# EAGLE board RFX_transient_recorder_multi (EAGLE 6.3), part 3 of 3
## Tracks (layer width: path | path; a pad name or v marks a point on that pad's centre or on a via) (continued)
N$84 (continued)
  Top 0.254: C72.2 52.8,19.14 55.9,19.14 55.9,20.14 56.1,20.34 57.7,20.34 57.7,19.04 IC4.2 57.8,18.94 R44.1 57.8,6.34 60.3,3.84 R43.2
N$85
  Top 0.254: R45.2 24.8,3.74 25.5,3.04 29.8,3.04 29.8,3.74 U2.1
N$86  (via drill 0.61 layers 1-2)
  Top 0.254: v33,6.84 29.1,6.84 26.1,3.84 R45.1 | v34.6,8.44 37,10.84 42,10.84 42,9.94 42.2,9.74 42.8,9.74 U1.22
  top_internal 0.254: v34.6,8.44 v33,6.84
N$87
  Top 0.254: R46.1 38.8,10.14 39.7,9.24 42.8,9.24 U1.23
N$88
  Top 0.254: 36.8,7.54 36.8,9.54 37.4,10.14 R46.2 | 36.8,7.54 36.8,4.44 37.4,3.84 R47.2 | 36.8,7.54 33.3,7.54 33.1,7.74 33.1,8.24 32.4,8.94 U2.6
N$89
  Top 0.254: R47.1 38.8,3.84 39,4.04 39,4.94 40.5,6.44 46.2,6.44 46.2,7.24 U1.29
N$90
  Top 0.254: U2.2 31.2,3.84 32.3,3.84 U2.3
N$91  (via drill 0.61 layers 1-2)
  Top 0.254: v40.6,11.84 36.5,11.84 33.7,9.04 U2.5 | v75.3,9.14 78.8,9.14 78.8,13.24 79,13.44 90.1,13.44 U3.2
  top_internal 0.254: v40.6,11.84 40.8,11.64 61.9,11.64 63.8,9.74 74.7,9.74 v75.3,9.14
N$92
  Top 0.254: R48.1 38.8,6.44 39.9,6.44 41.7,8.24 43.8,8.24 43.8,9.94 43.6,10.14 42.9,10.14 U1.21
N$93  (via drill 0.61 layers 1-2)
  Top 0.254: v38,7.44 38,6.94 37.5,6.44 R48.2 | v74.5,7.44 78.5,7.44 80.6,9.54 88.7,9.54 88.7,11.14 89.6,12.04 90.1,12.04 U3.3
  top_internal 0.254: v74.5,7.44 v38,7.44
N$94  (via drill 0.61 layers 1-2)
  Top 0.254: 55.9,4.94 55.9,3.34 55.4,2.84 50.7,2.84 50.7,5.74 50,6.44 49.3,6.44 49.3,7.24 U1.35 | 55.9,4.94 55.9,5.74 56.5,6.34 C74.2 | v75.3,5.64 78.6,5.64 79.3,6.34 R49.2 | 55.9,4.94 v56.6,4.94
  top_internal 0.254: v75.3,5.64 74.6,4.94 v56.6,4.94
N$95
  Top 0.254: R49.1 78.1,6.44 78.8,7.14 88.7,7.14 88.7,6.64 89.6,5.74 90.1,5.74 U16.6
N$96  (via drill 0.61 layers 1-2)
  Top 0.254: v48.3,5.84 48.7,6.24 48.7,7.24 U1.34 | v63,3.84 65,1.84 88.7,1.84 88.7,3.54 89.6,4.44 U16.7
  top_internal 0.254: v48.3,5.84 50.3,3.84 v63,3.84
N$97  (via drill 0.61 layers 1-2)
  Top 0.254: v103.8,8.54 103.8,9.94 99.8,13.94 R50.2 | v106.3,6.04 105.1,6.04 U17.5
  top_internal 0.254: v106.3,6.04 v103.8,8.54
N$98
  Top 0.254: R51.2 103.7,7.44 103.7,5.24 104.2,4.74 105,4.74 U17.7
N$99  (via drill 0.61 layers 1-2)
  Top 0.254: v98.4,12.84 98.4,13.94 R50.1 | v93.6,12.84 95.3,12.84 95.3,13.24 U3.7
  top_internal 0.254: v93.6,12.84 v98.4,12.84
N$100  (via drill 0.61 layers 1-2)
  Top 0.254: v98.4,10.34 98.4,11.34 R51.1 | v96.8,9.94 96.7,10.04 96.7,11.14 95.8,12.04 95.4,12.04 U3.6
  top_internal 0.254: v98.4,10.34 98,9.94 v96.8,9.94
N$101  (via drill 0.61 layers 1-2)
  Top 0.254: v113.8,2.54 R52.2 | v112.1,3.34 111.4,4.04 110.9,4.04 U17.9
  top_internal 0.254: v113.8,2.54 113,3.34 v112.1,3.34
N$102
  Top 0.254: 113.1,5.64 116.2,2.54 R52.1 | 113.1,5.64 113.1,10.84 111.9,12.04 U18.1 | U16.3 95.3,5.64 93.9,5.64 93.9,2.84 94.4,2.34 113,2.34 113,5.64 113.1,5.64
N$103  (via drill 0.61 layers 1-2)
  Top 0.254: v107.1,19.04 103.6,19.04 R53.1 | v96.8,7.84 96.8,4.54 95.4,4.54 U16.2
  top_internal 0.254: 107.65,18.49 110.9,15.24 X7.8 | 107.65,18.49 v107.1,19.04 | v96.8,7.84 98.5,9.54 98.7,9.54 107.65,18.49
N$104
  Top 0.254: U18.2 111.9,13.34 111.9,14.54 U18.3
N$105  (via drill 0.61)
  Top 0.254: 104.9,14.04 106.6,14.04 106.6,14.54 U18.6 | 104.9,14.04 103.6,14.04 R54.1 | v104.9,14.14 104.9,14.04
  bottom_internal 0.254: v104.9,14.14 124.4,14.14 124.4,15.24 X7.7
N$106  (via drill 0.61 layers 1-2)
  Top 0.254: 107.9,24.34 107.9,16.34 108,16.24 108,13.44 107.25,12.69 | 107.9,24.34 107.9,24.74 108.5,25.34 C81.2 | 107.25,12.69 106.7,12.14 U18.8 | v110.9,25.34 112,25.34 U19.5 | v108,24.34 107.9,24.34 | 107.25,12.69 106.7,13.24 U18.7
  top_internal 0.254: v110.9,25.34 109.9,24.34 v108,24.34
N$107  (via drill 0.61 layers 1-2)
  Top 0.254: v117.5,24.34 117.5,25.34 C82.2 | v114.8,24.54 114,25.34 U19.4
  top_internal 0.254: v117.5,24.34 117.3,24.54 v114.8,24.54
N$108  (via drill 0.61 layers 1-2)
  Top 0.254: v74.9,12.84 74.9,9.94 77.4,9.94 77.6,10.14 78,10.14 C54.1 | v66.8,20.94 64.8,20.94 64.8,20.04 U20.4
  top_internal 0.254: v66.8,20.94 v74.9,12.84
N$109  (via drill 0.61 layers 1-2)
  Top 0.254: v77.1,10.74 77.1,11.74 78,12.64 C55.1 | v67.6,10.64 66.1,10.64 66.1,9.84 U21.4
  top_internal 0.254: v77.1,10.74 77,10.64 v67.6,10.64
N$110
  Top 0.254: C56.1 49,24.14 49.3,24.44 49.3,25.74 49.5,25.94 64.7,25.94 64.7,25.14 U22.4
N$111
  Top 0.254: C57.1 73,8.84 69.9,5.74 69.9,2.74 69.5,2.34 65.1,2.34 65.1,3.84 66,4.74 U23.4
N$112  (via drill 0.61 layers 1-2)
  Top 0.254: v100.3,15.94 106.6,15.94 U18.5
  top_internal 0.254: v100.3,15.94 99.8,16.44 97.8,16.44 U24.P$14
N$115  (via drill 0.61 layers 1-2)
  Top 0.254: X6.9 24.1,17.84 24.1,20.24 X6.10 | U24.P$7 82.5,24.04 79.8,21.34 73.4,21.34 73.4,20.44 C2.1.- 73.4,20.24 72.2,19.04 72.2,14.94 69.6,14.94 69.5,14.84 68.8,14.84 IC3.3 68.7,14.84 68.7,14.04 IC3.2 68.8,14.04 69.5,13.34 69.5,12.04 v62.6,12.04
  top_internal 0.254: v62.6,12.04 58.4,12.04 53.9,16.54 25.4,16.54 24.2,17.74 X6.9
N$116  (via drill 0.61 layers 1-2)
  Top 0.254: X6.7 21.6,17.84 21.6,20.24 X6.8 21.7,20.34 26.6,25.24 v48.5,25.24 | U23.1 68.7,2.94 69.5,2.94 69.5,4.14 68.9,4.74 68.7,4.74 U23.3 68.7,4.84 68.7,7.94 U21.1 68.8,7.84 69.5,8.54 69.5,9.84 | 69.5,9.84 U21.3 | 68.2,18.14 67.4,18.14 U20.1 | 68.2,18.14 68.2,19.44 67.7,19.94 67.4,19.94 U20.3 67.7,20.04 67.7,22.44 | 67.7,22.44 67.7,22.84 67.4,23.14 U22.1 67.6,23.04 68.2,23.64 68.2,24.14 | 68.2,24.14 68.2,25.04 67.4,25.04 U22.3 | 68.2,24.14 73.4,24.14 C59.+ 73.5,24.24 73.5,25.74 83.4,25.74 85,24.14 U24.P$6 | v69.9,14.14 69.9,10.34 69.5,9.94 69.5,9.84 | v69.9,15.74 68.2,17.44 68.2,18.14 | 67.7,22.44 v60.4,22.44
  top_internal 0.254: v69.9,15.74 v69.9,14.14 | v48.5,25.24 51,22.74 60.1,22.74 v60.4,22.44
N$117  (via drill 0.61 layers 1-2)
  Top 0.254: v109.6,5.34 110.8,5.34 U17.11
  top_internal 0.254: v109.6,5.34 110.3,6.04 122.9,6.04 124.4,7.54 X7.1
N$118  (via drill 0.61 layers 1-2)
  Top 0.254: v112.3,6.84 112.3,6.04 110.9,6.04 U17.12
  top_internal 0.254: v112.3,6.84 113,7.54 121.9,7.54 X7.2
N$119  (via drill 0.61 layers 1-2)
  Top 0.254: v109.6,6.54 109.6,6.64 110.8,6.64 U17.13
  top_internal 0.254: v109.6,6.54 112.2,9.14 123.4,9.14 124.4,10.14 X7.3
N$120  (via drill 0.61 layers 1-2)
  Top 0.254: v109.3,7.74 109.3,7.34 110.8,7.34 U17.14
  top_internal 0.254: v109.3,7.74 111.7,10.14 121.9,10.14 X7.4
N$121  (via drill 0.61 layers 1-2)
  Top 0.254: v110,10.94 110,8.04 110.8,8.04 U17.15
  top_internal 0.254: v110,10.94 112.8,13.74 123.4,13.74 124.4,12.74 X7.5
N$122  (via drill 0.61)
  Top 0.254: v112.3,8.14 112.3,8.54 110.9,8.54 U17.16
  bottom_internal 0.254: v112.3,8.14 116.8,12.64 121.9,12.64 X7.6
N$123
  Top 0.254: R62.2 4.4,50.8 3.2,52 3.2,53.3 C86.1 3.2,53.4 3.2,55 5.3,57.1 L5.2
N$124
  Top 0.254: R58.1 3.2,64.7 3.2,61 C85.1 3.1,60.9 3.1,57.9 2.4,57.2 L5.1
N$125
  Top 0.254: C86.2 4.5,53.3 9.5,53.3 R63.2 9.6,53.4 9.6,55.1 11.6,57.1 L6.2
N$126
  Top 0.254: C85.2 4.5,61 8.2,61 R59.1 8.3,60.9 8.3,57.5 8.6,57.2 L6.1
N$127
  Top 0.254: 14.6,50.1 16.4,50.1 16.5,50.2 16.5,59.4 18.8,59.4 U$3.11 | 14.6,50.1 R65.1 14.6,50.9 14.6,53.3 R66.2 14.6,53.4 14.6,57.1 C87.1 | 14.6,50.1 3.9,50.1 3.2,50.8 R62.1
N$128  (via drill 0.61, 0.61 layers 1-2)
  Top 0.254: R64.1 10.8,53.3 R63.1 10.9,53.4 v13.7,56.2 | 23.8,59.4 24.2,59.4 24.2,59 24.7,58.5 R67.2 | 23.8,59.4 21.8,59.4 U$3.2 | v31.9,64 31.9,65.5 32.4,66 C88.1 | 23.8,59.4 v23.8,59.1
  top_internal 0.254: v13.7,56.2 16.6,59.1 v23.8,59.1
  bottom_internal 0.254: v31.9,64 27,59.1 v23.8,59.1
N$129
  Top 0.254: X8.3 16.5,66 14.8,64.3 14.8,62.4 13.4,61 R57.2 13.3,60.9 13.3,60.2 9.1,60.2 8.9,60.4 8.9,61.7 7.5,61.7 4.5,64.7 R58.2
N$130
  Top 0.254: R59.2 9.6,61 12,61 R57.1 12,61.1 14.4,63.5 14.4,65 15.5,66.1 15.5,67.5 16.5,68.5 X8.4
N$131
  Top 0.254: R66.1 15.9,53.4 15.9,57.1 C87.2 15.9,57.2 15.9,60 | 15.9,60 18.8,60 U$3.10 | 15.9,60 15.9,60.9 R68.2
N$132  (via drill 0.61 layers 1-2)
  Top 0.254: C88.2 31.1,63.1 | 31.1,63.1 R69.2 | 26.7,62.8 25,62.8 24,61.8 24,59.9 21.8,59.9 U$3.3 | 26.7,62.8 26.7,60.4 26.1,59.8 26.1,58.5 R67.1 | v30.3,63.1 31.1,63.1 | v28.3,63 26.7,63 26.7,62.8
  top_internal 0.254: v30.3,63.1 30.2,63 v28.3,63
N$133  (via drill 0.61 layers 1-2)
  Top 0.254: R68.1 18,61.8 v18,62 | v25.3,62 26,61.3 26,61 C89.2 | v52.3,57.9 51.1,57.9 U25.39
  top_internal 0.254: v18,62 v25.3,62 26.1,62 28.8,59.3 50.9,59.3 v52.3,57.9
N$134  (via drill 0.61)
  Top 0.254: R69.1 32.4,60.9 | 32.4,60.9 32.4,59 31.8,58.4 31.8,55.8 26.1,55.8 C90.2 | v52.3,59.1 52.3,59.9 51.1,59.9 U25.43 | 32.4,60.9 v38.6,60.9
  bottom_internal 0.254: v52.3,59.1 50.5,60.9 v38.6,60.9
N$135  (via drill 0.61 layers 1-2)
  Top 0.254: v60.7,61.1 60.7,61.9 60.4,62.2 R61.1 | v62.6,62.1 66,62.1 66,63.1 IC5.4 | v70.7,61.5 71.1,61.5 72.6,63 72.6,64.3 73,64.7 R60.1
  top_internal 0.254: v60.7,61.1 61.7,62.1 v62.6,62.1 67.4,62.1 67.9,61.6 70.6,61.6 v70.7,61.5
N$136  (via drill 0.61 layers 1-2)
  Top 0.254: IC6.6 59,72.5 57.8,72.5 IC6.7 58,72.4 58,69.9 57.1,69 50.8,69 v50.3,68.5 | v18.8,61.2 18.8,60.5 U$3.9 | v21.9,61.2 21.8,61.1 21.8,60.5 U$3.4 | 30.55,67.95 30.5,67.9 30.5,64.4 29.5,63.4 29.5,61.5 v27.5,59.5 | 30.55,67.95 31.1,68.5 C91.2 | v37.9,68.4 33,68.4 33,68 32.9,67.9 30.6,67.9 30.55,67.95
  top_internal 0.254: v18.8,61.2 v21.9,61.2 22,61.2 22.3,61.5 23.3,61.5 23.6,61.2 25.8,61.2 v27.5,59.5 | v50.3,68.5 50.2,68.4 v37.9,68.4
N$137  (via drill 0.61 layers 1-2)
  Top 0.254: v56.6,51 56.6,52 R70.2 | v58.2,51 61.6,51 61.6,52 R71.1 61.7,52.1 61.7,52.5 62.2,53 62.2,58.6 | C103.1 62.2,59.1 62.2,58.6 | v59.5,58.8 59.5,64 59.6,64.1 59.6,71.7 60.3,72.4 IC6.5 | 62.2,58.6 v61.8,58.6
  top_internal 0.254: v58.2,51 v56.6,51 | v59.5,58.8 59.7,58.6 v61.8,58.6
N$138
  Top 0.254: R70.1 55.2,52.1 52.3,52.1 C104.+ 52.3,55.7 51.1,56.9 U25.37
N$139
  Top 0.254: C105.1 55.2,62.2 52,62.2 52,61.7 51.8,61.5 51.1,61.5 U25.46
N$140  (via drill 0.61 layers 1-2)
  Top 0.254: R72.2 56.5,67.2 IC6.1 56.4,66.6 52.2,66.6 51.5,67.3 C114.1 51.3,67.3 v49.9,67.3 | 15.2,59.1 15.3,59.1 15.3,51.3 15.8,50.8 R65.2 | 15.2,59.1 14.2,59.1 13.6,58.5 13.6,57.3 10.2,53.9 10.2,51.4 9.6,50.8 R64.2 | v27.3,67.6 22.5,62.8 15.2,62.8 15.2,59.1
  top_internal 0.254: v49.9,67.3 49.6,67.6 v27.3,67.6
N$141
  Top 0.254: C114.2 52.8,67.4 55.9,67.4 55.9,68.4 56.1,68.6 57.7,68.6 57.7,67.3 IC6.2 57.8,67.2 R72.1 57.8,54.6 60.3,52.1 R71.2
N$142
  Top 0.254: R73.2 24.8,52 25.5,51.3 29.8,51.3 29.8,52 U26.1
N$143  (via drill 0.61 layers 1-2)
  Top 0.254: v33,55.1 29.1,55.1 26.1,52.1 R73.1 | v34.6,56.7 37,59.1 42,59.1 42,58.2 42.2,58 42.8,58 U25.22
  top_internal 0.254: v34.6,56.7 v33,55.1
N$144
  Top 0.254: R74.1 38.8,58.4 39.7,57.5 42.8,57.5 U25.23
N$145
  Top 0.254: 36.8,55.8 36.8,57.8 37.4,58.4 R74.2 | 36.8,55.8 36.8,52.7 37.4,52.1 R75.2 | 36.8,55.8 33.3,55.8 33.1,56 33.1,56.5 32.4,57.2 U26.6
N$146
  Top 0.254: R75.1 38.8,52.1 39,52.3 39,53.2 40.5,54.7 46.2,54.7 46.2,55.5 U25.29
N$147
  Top 0.254: U26.2 31.2,52.1 32.3,52.1 U26.3
N$148  (via drill 0.61 layers 1-2)
  Top 0.254: v40.6,60.1 36.5,60.1 33.7,57.3 U26.5 | v75.3,57.4 78.8,57.4 78.8,61.5 79,61.7 90.1,61.7 U27.2
  top_internal 0.254: v40.6,60.1 40.8,59.9 61.9,59.9 63.8,58 74.7,58 v75.3,57.4
N$149
  Top 0.254: R76.1 38.8,54.7 39.9,54.7 41.7,56.5 43.8,56.5 43.8,58.2 43.6,58.4 42.9,58.4 U25.21
N$150  (via drill 0.61 layers 1-2)
  Top 0.254: v38,55.7 38,55.2 37.5,54.7 R76.2 | v74.5,55.7 78.5,55.7 80.6,57.8 88.7,57.8 88.7,59.4 89.6,60.3 90.1,60.3 U27.3
  top_internal 0.254: v74.5,55.7 v38,55.7
N$151  (via drill 0.61 layers 1-2)
  Top 0.254: 55.9,53.2 55.9,51.6 55.4,51.1 50.7,51.1 50.7,54 50,54.7 49.3,54.7 49.3,55.5 U25.35 | 55.9,53.2 55.9,54 56.5,54.6 C116.2 | v75.3,53.9 78.6,53.9 79.3,54.6 R77.2 | 55.9,53.2 v56.6,53.2
  top_internal 0.254: v75.3,53.9 74.6,53.2 v56.6,53.2
N$152
  Top 0.254: R77.1 78.1,54.7 78.8,55.4 88.7,55.4 88.7,54.9 89.6,54 90.1,54 U28.6
N$153  (via drill 0.61 layers 1-2)
  Top 0.254: v48.3,54.1 48.7,54.5 48.7,55.5 U25.34 | v63,52.1 65,50.1 88.7,50.1 88.7,51.8 89.6,52.7 U28.7
  top_internal 0.254: v48.3,54.1 50.3,52.1 v63,52.1
N$154  (via drill 0.61 layers 1-2)
  Top 0.254: v103.8,56.8 103.8,58.2 99.8,62.2 R78.2 | v106.3,54.3 105.1,54.3 U29.5
  top_internal 0.254: v106.3,54.3 v103.8,56.8
N$155
  Top 0.254: R79.2 103.7,55.7 103.7,53.5 104.2,53 105,53 U29.7
N$156  (via drill 0.61 layers 1-2)
  Top 0.254: v98.4,61.1 98.4,62.2 R78.1 | v93.6,61.1 95.3,61.1 95.3,61.5 U27.7
  top_internal 0.254: v93.6,61.1 v98.4,61.1
N$157  (via drill 0.61 layers 1-2)
  Top 0.254: v98.4,58.6 98.4,59.6 R79.1 | v96.8,58.2 96.7,58.3 96.7,59.4 95.8,60.3 95.4,60.3 U27.6
  top_internal 0.254: v98.4,58.6 98,58.2 v96.8,58.2
N$158  (via drill 0.61 layers 1-2)
  Top 0.254: v113.8,50.8 R80.2 | v112.1,51.6 111.4,52.3 110.9,52.3 U29.9
  top_internal 0.254: v113.8,50.8 113,51.6 v112.1,51.6
N$159
  Top 0.254: 113.1,53.9 116.2,50.8 R80.1 | 113.1,53.9 113.1,59.1 111.9,60.3 U30.1 | U28.3 95.3,53.9 93.9,53.9 93.9,51.1 94.4,50.6 113,50.6 113,53.9 113.1,53.9
N$160  (via drill 0.61 layers 1-2)
  Top 0.254: v107.1,67.3 103.6,67.3 R81.1 | v96.8,56.1 96.8,52.8 95.4,52.8 U28.2
  top_internal 0.254: 107.65,66.75 110.9,63.5 X9.8 | 107.65,66.75 v107.1,67.3 | v96.8,56.1 98.5,57.8 98.7,57.8 107.65,66.75
N$161
  Top 0.254: U30.2 111.9,61.6 111.9,62.8 U30.3
N$162  (via drill 0.61)
  Top 0.254: 104.9,62.3 106.6,62.3 106.6,62.8 U30.6 | 104.9,62.3 103.6,62.3 R82.1 | v104.9,62.4 104.9,62.3
  bottom_internal 0.254: v104.9,62.4 124.4,62.4 124.4,63.5 X9.7
N$163  (via drill 0.61 layers 1-2)
  Top 0.254: 107.9,72.6 107.9,64.6 108,64.5 108,61.7 107.25,60.95 | 107.9,72.6 107.9,73 108.5,73.6 C123.2 | 107.25,60.95 106.7,60.4 U30.8 | v110.9,73.6 112,73.6 U31.5 | v108,72.6 107.9,72.6 | 107.25,60.95 106.7,61.5 U30.7
  top_internal 0.254: v110.9,73.6 109.9,72.6 v108,72.6
N$164  (via drill 0.61 layers 1-2)
  Top 0.254: v117.5,72.6 117.5,73.6 C124.2 | v114.8,72.8 114,73.6 U31.4
  top_internal 0.254: v117.5,72.6 117.3,72.8 v114.8,72.8
N$165  (via drill 0.61 layers 1-2)
  Top 0.254: v74.9,61.1 74.9,58.2 77.4,58.2 77.6,58.4 78,58.4 C96.1 | v66.8,69.2 64.8,69.2 64.8,68.3 U32.4
  top_internal 0.254: v66.8,69.2 v74.9,61.1
N$166  (via drill 0.61 layers 1-2)
  Top 0.254: v77.1,59 77.1,60 78,60.9 C97.1 | v67.6,58.9 66.1,58.9 66.1,58.1 U33.4
  top_internal 0.254: v77.1,59 77,58.9 v67.6,58.9
N$167
  Top 0.254: C98.1 49,72.4 49.3,72.7 49.3,74 49.5,74.2 64.7,74.2 64.7,73.4 U34.4
N$168
  Top 0.254: C99.1 73,57.1 69.9,54 69.9,51 69.5,50.6 65.1,50.6 65.1,52.1 66,53 U35.4
N$169  (via drill 0.61 layers 1-2)
  Top 0.254: v100.3,64.2 106.6,64.2 U30.5
  top_internal 0.254: v100.3,64.2 99.8,64.7 97.8,64.7 U36.P$14
N$172  (via drill 0.61 layers 1-2)
  Top 0.254: X8.9 24.1,66.1 24.1,68.5 X8.10 | U36.P$7 82.5,72.3 79.8,69.6 73.4,69.6 73.4,68.7 C2.2.- 73.4,68.5 72.2,67.3 72.2,63.2 69.6,63.2 69.5,63.1 68.8,63.1 IC5.3 68.7,63.1 68.7,62.3 IC5.2 68.8,62.3 69.5,61.6 69.5,60.3 v62.6,60.3
  top_internal 0.254: v62.6,60.3 58.4,60.3 53.9,64.8 25.4,64.8 24.2,66 X8.9
N$173  (via drill 0.61 layers 1-2)
  Top 0.254: X8.7 21.6,66.1 21.6,68.5 X8.8 21.7,68.6 26.6,73.5 v48.5,73.5 | U35.1 68.7,51.2 69.5,51.2 69.5,52.4 68.9,53 68.7,53 U35.3 68.7,53.1 68.7,56.2 U33.1 68.8,56.1 69.5,56.8 69.5,58.1 | 69.5,58.1 U33.3 | 68.2,66.4 67.4,66.4 U32.1 | 68.2,66.4 68.2,67.7 67.7,68.2 67.4,68.2 U32.3 67.7,68.3 67.7,70.7 | 67.7,70.7 67.7,71.1 67.4,71.4 U34.1 67.6,71.3 68.2,71.9 68.2,72.4 | 68.2,72.4 68.2,73.3 67.4,73.3 U34.3 | 68.2,72.4 73.4,72.4 C101.+ 73.5,72.5 73.5,74 83.4,74 85,72.4 U36.P$6 | v69.9,62.4 69.9,58.6 69.5,58.2 69.5,58.1 | v69.9,64 68.2,65.7 68.2,66.4 | 67.7,70.7 v60.4,70.7
  top_internal 0.254: v69.9,64 v69.9,62.4 | v48.5,73.5 51,71 60.1,71 v60.4,70.7
N$174  (via drill 0.61 layers 1-2)
  Top 0.254: v109.6,53.6 110.8,53.6 U29.11
  top_internal 0.254: v109.6,53.6 110.3,54.3 122.9,54.3 124.4,55.8 X9.1
N$175  (via drill 0.61 layers 1-2)
  Top 0.254: v112.3,55.1 112.3,54.3 110.9,54.3 U29.12
  top_internal 0.254: v112.3,55.1 113,55.8 121.9,55.8 X9.2
N$176  (via drill 0.61 layers 1-2)
  Top 0.254: v109.6,54.8 109.6,54.9 110.8,54.9 U29.13
  top_internal 0.254: v109.6,54.8 112.2,57.4 123.4,57.4 124.4,58.4 X9.3
N$177  (via drill 0.61 layers 1-2)
  Top 0.254: v109.3,56 109.3,55.6 110.8,55.6 U29.14
  top_internal 0.254: v109.3,56 111.7,58.4 121.9,58.4 X9.4
N$178  (via drill 0.61 layers 1-2)
  Top 0.254: v110,59.2 110,56.3 110.8,56.3 U29.15
  top_internal 0.254: v110,59.2 112.8,62 123.4,62 124.4,61 X9.5
N$179  (via drill 0.61)
  Top 0.254: v112.3,56.4 112.3,56.8 110.9,56.8 U29.16
  bottom_internal 0.254: v112.3,56.4 116.8,60.9 121.9,60.9 X9.6
N$180
  Top 0.254: R90.2 4.4,26.67 3.2,27.87 3.2,29.17 C128.1 3.2,29.27 3.2,30.87 5.3,32.97 L7.2
N$181
  Top 0.254: R86.1 3.2,40.57 3.2,36.87 C127.1 3.1,36.77 3.1,33.77 2.4,33.07 L7.1
N$182
  Top 0.254: C128.2 4.5,29.17 9.5,29.17 R91.2 9.6,29.27 9.6,30.97 11.6,32.97 L8.2
N$183
  Top 0.254: C127.2 4.5,36.87 8.2,36.87 R87.1 8.3,36.77 8.3,33.37 8.6,33.07 L8.1
N$184
  Top 0.254: 14.6,25.97 16.4,25.97 16.5,26.07 16.5,35.27 18.8,35.27 U$4.11 | 14.6,25.97 R93.1 14.6,26.77 14.6,29.17 R94.2 14.6,29.27 14.6,32.97 C129.1 | 14.6,25.97 3.9,25.97 3.2,26.67 R90.1
N$185  (via drill 0.61, 0.61 layers 1-2)
  Top 0.254: R92.1 10.8,29.17 R91.1 10.9,29.27 v13.7,32.07 | 23.8,35.27 24.2,35.27 24.2,34.87 24.7,34.37 R95.2 | 23.8,35.27 21.8,35.27 U$4.2 | v31.9,39.87 31.9,41.37 32.4,41.87 C130.1 | 23.8,35.27 v23.8,34.97
  top_internal 0.254: v13.7,32.07 16.6,34.97 v23.8,34.97
  bottom_internal 0.254: v31.9,39.87 27,34.97 v23.8,34.97
N$186
  Top 0.254: X10.3 16.5,41.87 14.8,40.17 14.8,38.27 13.4,36.87 R85.2 13.3,36.77 13.3,36.07 9.1,36.07 8.9,36.27 8.9,37.57 7.5,37.57 4.5,40.57 R86.2
N$187
  Top 0.254: R87.2 9.6,36.87 12,36.87 R85.1 12,36.97 14.4,39.37 14.4,40.87 15.5,41.97 15.5,43.37 16.5,44.37 X10.4
N$188
  Top 0.254: R94.1 15.9,29.27 15.9,32.97 C129.2 15.9,33.07 15.9,35.87 | 15.9,35.87 18.8,35.87 U$4.10 | 15.9,35.87 15.9,36.77 R96.2
N$189  (via drill 0.61 layers 1-2)
  Top 0.254: C130.2 31.1,38.97 | 31.1,38.97 R97.2 | 26.7,38.67 25,38.67 24,37.67 24,35.77 21.8,35.77 U$4.3 | 26.7,38.67 26.7,36.27 26.1,35.67 26.1,34.37 R95.1 | v30.3,38.97 31.1,38.97 | v28.3,38.87 26.7,38.87 26.7,38.67
  top_internal 0.254: v30.3,38.97 30.2,38.87 v28.3,38.87
N$190  (via drill 0.61 layers 1-2)
  Top 0.254: R96.1 18,37.67 v18,37.87 | v25.3,37.87 26,37.17 26,36.87 C131.2 | v52.3,33.77 51.1,33.77 U37.39
  top_internal 0.254: v18,37.87 v25.3,37.87 26.1,37.87 28.8,35.17 50.9,35.17 v52.3,33.77
N$191  (via drill 0.61)
  Top 0.254: R97.1 32.4,36.77 | 32.4,36.77 32.4,34.87 31.8,34.27 31.8,31.67 26.1,31.67 C132.2 | v52.3,34.97 52.3,35.77 51.1,35.77 U37.43 | 32.4,36.77 v38.6,36.77
  bottom_internal 0.254: v52.3,34.97 50.5,36.77 v38.6,36.77
N$192  (via drill 0.61 layers 1-2)
  Top 0.254: v60.7,36.97 60.7,37.77 60.4,38.07 R89.1 | v62.6,37.97 66,37.97 66,38.97 IC7.4 | v70.7,37.37 71.1,37.37 72.6,38.87 72.6,40.17 73,40.57 R88.1
  top_internal 0.254: v60.7,36.97 61.7,37.97 v62.6,37.97 67.4,37.97 67.9,37.47 70.6,37.47 v70.7,37.37
N$193  (via drill 0.61 layers 1-2)
  Top 0.254: IC8.6 59,48.37 57.8,48.37 IC8.7 58,48.27 58,45.77 57.1,44.87 50.8,44.87 v50.3,44.37 | v18.8,37.07 18.8,36.37 U$4.9 | v21.9,37.07 21.8,36.97 21.8,36.37 U$4.4 | 30.55,43.82 30.5,43.77 30.5,40.27 29.5,39.27 29.5,37.37 v27.5,35.37 | 30.55,43.82 31.1,44.37 C133.2 | v37.9,44.27 33,44.27 33,43.87 32.9,43.77 30.6,43.77 30.55,43.82
  top_internal 0.254: v18.8,37.07 v21.9,37.07 22,37.07 22.3,37.37 23.3,37.37 23.6,37.07 25.8,37.07 v27.5,35.37 | v50.3,44.37 50.2,44.27 v37.9,44.27
N$194  (via drill 0.61 layers 1-2)
  Top 0.254: v56.6,26.87 56.6,27.87 R98.2 | v58.2,26.87 61.6,26.87 61.6,27.87 R99.1 61.7,27.97 61.7,28.37 62.2,28.87 62.2,34.47 | C145.1 62.2,34.97 62.2,34.47 | v59.5,34.67 59.5,39.87 59.6,39.97 59.6,47.57 60.3,48.27 IC8.5 | 62.2,34.47 v61.8,34.47
  top_internal 0.254: v58.2,26.87 v56.6,26.87 | v59.5,34.67 59.7,34.47 v61.8,34.47
N$195
  Top 0.254: R98.1 55.2,27.97 52.3,27.97 C146.+ 52.3,31.57 51.1,32.77 U37.37
N$196
  Top 0.254: C147.1 55.2,38.07 52,38.07 52,37.57 51.8,37.37 51.1,37.37 U37.46
N$197  (via drill 0.61 layers 1-2)
  Top 0.254: R100.2 56.5,43.07 IC8.1 56.4,42.47 52.2,42.47 51.5,43.17 C156.1 51.3,43.17 v49.9,43.17 | 15.2,34.97 15.3,34.97 15.3,27.17 15.8,26.67 R93.2 | 15.2,34.97 14.2,34.97 13.6,34.37 13.6,33.17 10.2,29.77 10.2,27.27 9.6,26.67 R92.2 | v27.3,43.47 22.5,38.67 15.2,38.67 15.2,34.97
  top_internal 0.254: v49.9,43.17 49.6,43.47 v27.3,43.47
N$198
  Top 0.254: C156.2 52.8,43.27 55.9,43.27 55.9,44.27 56.1,44.47 57.7,44.47 57.7,43.17 IC8.2 57.8,43.07 R100.1 57.8,30.47 60.3,27.97 R99.2
N$199
  Top 0.254: R101.2 24.8,27.87 25.5,27.17 29.8,27.17 29.8,27.87 U38.1
N$200  (via drill 0.61 layers 1-2)
  Top 0.254: v33,30.97 29.1,30.97 26.1,27.97 R101.1 | v34.6,32.57 37,34.97 42,34.97 42,34.07 42.2,33.87 42.8,33.87 U37.22
  top_internal 0.254: v34.6,32.57 v33,30.97
N$201
  Top 0.254: R102.1 38.8,34.27 39.7,33.37 42.8,33.37 U37.23
N$202
  Top 0.254: 36.8,31.67 36.8,33.67 37.4,34.27 R102.2 | 36.8,31.67 36.8,28.57 37.4,27.97 R103.2 | 36.8,31.67 33.3,31.67 33.1,31.87 33.1,32.37 32.4,33.07 U38.6
N$203
  Top 0.254: R103.1 38.8,27.97 39,28.17 39,29.07 40.5,30.57 46.2,30.57 46.2,31.37 U37.29
N$204
  Top 0.254: U38.2 31.2,27.97 32.3,27.97 U38.3
N$205  (via drill 0.61 layers 1-2)
  Top 0.254: v40.6,35.97 36.5,35.97 33.7,33.17 U38.5 | v75.3,33.27 78.8,33.27 78.8,37.37 79,37.57 90.1,37.57 U39.2
  top_internal 0.254: v40.6,35.97 40.8,35.77 61.9,35.77 63.8,33.87 74.7,33.87 v75.3,33.27
N$206
  Top 0.254: R104.1 38.8,30.57 39.9,30.57 41.7,32.37 43.8,32.37 43.8,34.07 43.6,34.27 42.9,34.27 U37.21
N$207  (via drill 0.61 layers 1-2)
  Top 0.254: v38,31.57 38,31.07 37.5,30.57 R104.2 | v74.5,31.57 78.5,31.57 80.6,33.67 88.7,33.67 88.7,35.27 89.6,36.17 90.1,36.17 U39.3
  top_internal 0.254: v74.5,31.57 v38,31.57
N$208  (via drill 0.61 layers 1-2)
  Top 0.254: 55.9,29.07 55.9,27.47 55.4,26.97 50.7,26.97 50.7,29.87 50,30.57 49.3,30.57 49.3,31.37 U37.35 | 55.9,29.07 55.9,29.87 56.5,30.47 C158.2 | v75.3,29.77 78.6,29.77 79.3,30.47 R105.2 | 55.9,29.07 v56.6,29.07
  top_internal 0.254: v75.3,29.77 74.6,29.07 v56.6,29.07
N$209
  Top 0.254: R105.1 78.1,30.57 78.8,31.27 88.7,31.27 88.7,30.77 89.6,29.87 90.1,29.87 U40.6
N$210  (via drill 0.61 layers 1-2)
  Top 0.254: v48.3,29.97 48.7,30.37 48.7,31.37 U37.34 | v63,27.97 65,25.97 88.7,25.97 88.7,27.67 89.6,28.57 U40.7
  top_internal 0.254: v48.3,29.97 50.3,27.97 v63,27.97
N$211  (via drill 0.61 layers 1-2)
  Top 0.254: v103.8,32.67 103.8,34.07 99.8,38.07 R106.2 | v106.3,30.17 105.1,30.17 U41.5
  top_internal 0.254: v106.3,30.17 v103.8,32.67
N$212
  Top 0.254: R107.2 103.7,31.57 103.7,29.37 104.2,28.87 105,28.87 U41.7
N$213  (via drill 0.61 layers 1-2)
  Top 0.254: v98.4,36.97 98.4,38.07 R106.1 | v93.6,36.97 95.3,36.97 95.3,37.37 U39.7
  top_internal 0.254: v93.6,36.97 v98.4,36.97
N$214  (via drill 0.61 layers 1-2)
  Top 0.254: v98.4,34.47 98.4,35.47 R107.1 | v96.8,34.07 96.7,34.17 96.7,35.27 95.8,36.17 95.4,36.17 U39.6
  top_internal 0.254: v98.4,34.47 98,34.07 v96.8,34.07
N$215  (via drill 0.61 layers 1-2)
  Top 0.254: v113.8,26.67 R108.2 | v112.1,27.47 111.4,28.17 110.9,28.17 U41.9
  top_internal 0.254: v113.8,26.67 113,27.47 v112.1,27.47
N$216
  Top 0.254: 113.1,29.77 116.2,26.67 R108.1 | 113.1,29.77 113.1,34.97 111.9,36.17 U42.1 | U40.3 95.3,29.77 93.9,29.77 93.9,26.97 94.4,26.47 113,26.47 113,29.77 113.1,29.77
N$217  (via drill 0.61 layers 1-2)
  Top 0.254: v107.1,43.17 103.6,43.17 R109.1 | v96.8,31.97 96.8,28.67 95.4,28.67 U40.2
  top_internal 0.254: 107.65,42.62 110.9,39.37 X11.8 | 107.65,42.62 v107.1,43.17 | v96.8,31.97 98.5,33.67 98.7,33.67 107.65,42.62
N$218
  Top 0.254: U42.2 111.9,37.47 111.9,38.67 U42.3
N$219  (via drill 0.61)
  Top 0.254: 104.9,38.17 106.6,38.17 106.6,38.67 U42.6 | 104.9,38.17 103.6,38.17 R110.1 | v104.9,38.27 104.9,38.17
  bottom_internal 0.254: v104.9,38.27 124.4,38.27 124.4,39.37 X11.7
N$220  (via drill 0.61 layers 1-2)
  Top 0.254: 107.9,48.47 107.9,40.47 108,40.37 108,37.57 107.25,36.82 | 107.9,48.47 107.9,48.87 108.5,49.47 C165.2 | 107.25,36.82 106.7,36.27 U42.8 | v110.9,49.47 112,49.47 U43.5 | v108,48.47 107.9,48.47 | 107.25,36.82 106.7,37.37 U42.7
  top_internal 0.254: v110.9,49.47 109.9,48.47 v108,48.47
N$221  (via drill 0.61 layers 1-2)
  Top 0.254: v117.5,48.47 117.5,49.47 C166.2 | v114.8,48.67 114,49.47 U43.4
  top_internal 0.254: v117.5,48.47 117.3,48.67 v114.8,48.67
N$222  (via drill 0.61 layers 1-2)
  Top 0.254: v74.9,36.97 74.9,34.07 77.4,34.07 77.6,34.27 78,34.27 C138.1 | v66.8,45.07 64.8,45.07 64.8,44.17 U44.4
  top_internal 0.254: v66.8,45.07 v74.9,36.97
N$223  (via drill 0.61 layers 1-2)
  Top 0.254: v77.1,34.87 77.1,35.87 78,36.77 C139.1 | v67.6,34.77 66.1,34.77 66.1,33.97 U45.4
  top_internal 0.254: v77.1,34.87 77,34.77 v67.6,34.77
N$224
  Top 0.254: C140.1 49,48.27 49.3,48.57 49.3,49.87 49.5,50.07 64.7,50.07 64.7,49.27 U46.4
N$225
  Top 0.254: C141.1 73,32.97 69.9,29.87 69.9,26.87 69.5,26.47 65.1,26.47 65.1,27.97 66,28.87 U47.4
N$226  (via drill 0.61 layers 1-2)
  Top 0.254: v100.3,40.07 106.6,40.07 U42.5
  top_internal 0.254: v100.3,40.07 99.8,40.57 97.8,40.57 U48.P$14
N$229  (via drill 0.61 layers 1-2)
  Top 0.254: X10.9 24.1,41.97 24.1,44.37 X10.10 | U48.P$7 82.5,48.17 79.8,45.47 73.4,45.47 73.4,44.57 C2.3.- 73.4,44.37 72.2,43.17 72.2,39.07 69.6,39.07 69.5,38.97 68.8,38.97 IC7.3 68.7,38.97 68.7,38.17 IC7.2 68.8,38.17 69.5,37.47 69.5,36.17 v62.6,36.17
  top_internal 0.254: v62.6,36.17 58.4,36.17 53.9,40.67 25.4,40.67 24.2,41.87 X10.9
N$230  (via drill 0.61 layers 1-2)
  Top 0.254: X10.7 21.6,41.97 21.6,44.37 X10.8 21.7,44.47 26.6,49.37 v48.5,49.37 | U47.1 68.7,27.07 69.5,27.07 69.5,28.27 68.9,28.87 68.7,28.87 U47.3 68.7,28.97 68.7,32.07 U45.1 68.8,31.97 69.5,32.67 69.5,33.97 | 69.5,33.97 U45.3 | 68.2,42.27 67.4,42.27 U44.1 | 68.2,42.27 68.2,43.57 67.7,44.07 67.4,44.07 U44.3 67.7,44.17 67.7,46.57 | 67.7,46.57 67.7,46.97 67.4,47.27 U46.1 67.6,47.17 68.2,47.77 68.2,48.27 | 68.2,48.27 68.2,49.17 67.4,49.17 U46.3 | 68.2,48.27 73.4,48.27 C143.+ 73.5,48.37 73.5,49.87 83.4,49.87 85,48.27 U48.P$6 | v69.9,38.27 69.9,34.47 69.5,34.07 69.5,33.97 | v69.9,39.87 68.2,41.57 68.2,42.27 | 67.7,46.57 v60.4,46.57
  top_internal 0.254: v69.9,39.87 v69.9,38.27 | v48.5,49.37 51,46.87 60.1,46.87 v60.4,46.57
N$231  (via drill 0.61 layers 1-2)
  Top 0.254: v109.6,29.47 110.8,29.47 U41.11
  top_internal 0.254: v109.6,29.47 110.3,30.17 122.9,30.17 124.4,31.67 X11.1
N$232  (via drill 0.61 layers 1-2)
  Top 0.254: v112.3,30.97 112.3,30.17 110.9,30.17 U41.12
  top_internal 0.254: v112.3,30.97 113,31.67 121.9,31.67 X11.2
N$233  (via drill 0.61 layers 1-2)
  Top 0.254: v109.6,30.67 109.6,30.77 110.8,30.77 U41.13
  top_internal 0.254: v109.6,30.67 112.2,33.27 123.4,33.27 124.4,34.27 X11.3
N$234  (via drill 0.61 layers 1-2)
  Top 0.254: v109.3,31.87 109.3,31.47 110.8,31.47 U41.14
  top_internal 0.254: v109.3,31.87 111.7,34.27 121.9,34.27 X11.4
N$235  (via drill 0.61 layers 1-2)
  Top 0.254: v110,35.07 110,32.17 110.8,32.17 U41.15
  top_internal 0.254: v110,35.07 112.8,37.87 123.4,37.87 124.4,36.87 X11.5
N$236  (via drill 0.61)
  Top 0.254: v112.3,32.27 112.3,32.67 110.9,32.67 U41.16
  bottom_internal 0.254: v112.3,32.27 116.8,36.77 121.9,36.77 X11.6

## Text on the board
tNames: FPGA area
